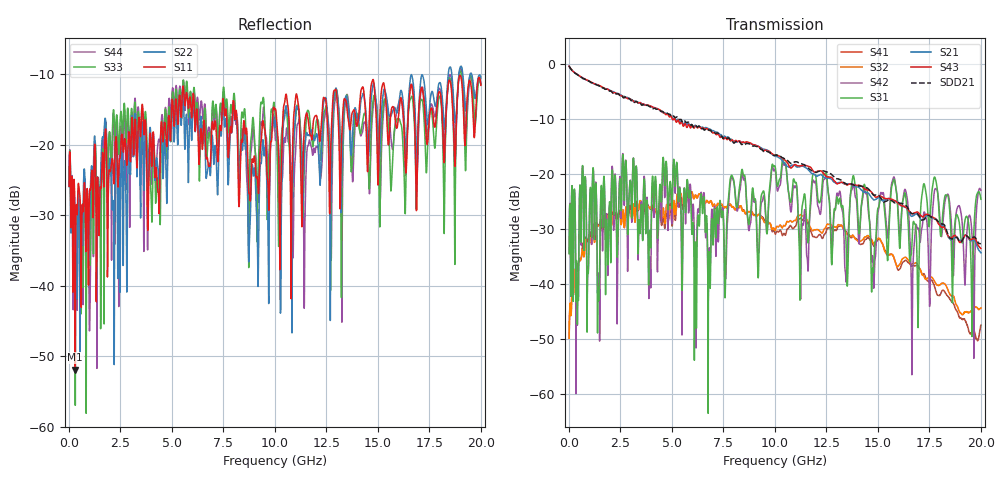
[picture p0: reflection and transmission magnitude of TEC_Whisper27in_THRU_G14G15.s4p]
! Tyco Electronics
! G14G15_THRU
!! PART DESCRIPTION: Whisper 27in Megtron 6 VLP-HVLP-VLP Channel Model, bulkhead 2.4mm test pts
!! MODEL DESCRIPTION: System 4-port S-parameter
!! MODEL STATUS: Measured
!! MODEL GEOMETRY: Channel Model
!! MODEL FREQUENCY RANGE: DC to 20.000 GHz in 10.000 MHz frequency steps
!! MODEL EDGE RATE LIMITATION: 25.00 ps (Using conservative 0.5/Fmax rule of thumb)
!! TIME-DOMAIN TRANSFORM CAUTIONS:
!! 1.) Do not simulate transient edge rates faster than the number listed above.  Edge rates faster than this number
!!  contain significant spectral content at frequencies above the model's highest frequency.
!! 2.) Even when simulating edge rates that are slower than the number listed above, be aware that the best time
!!  resolution possible with a direct iFFT is (1 / 2Fmax).  As a result, time resolution is typically not adequate
!!  for most time-domain simulations unless tricks such as windowing are used to minimize leakage and aliasing.
!! 3.) Because the model has a uniform frequency step, a direct iFFT will result in an impulse that that has a time
!!  length given by either (1 / Fstep) or (1 / 2Fstep), depending on the transform being used.  Care has been taken
!!  in selecting the frequency step to ensure a settled impulse response for the model.  Therefore, convolution with
!!  the model's impulse response should present no issues.  However, if directly concatenating s-parameter models
!!  in the frequency domain a user must either interpolate necessary interim frequencies or complete impulse response
!!  zero-padding.  Impulse response zero-padding is more difficult, but more accurate.
!! PORT DEFINITIONS:
!! Port  1  ----->  Side A  G14  Side B  <-----  Port  2
!! Port  3  ----->  Side A  G15  Side B  <-----  Port  4
! Point-to-Point link (differential)  !
! Connectors:  !
!  1: STRADA Whisper  !
! Materials:  !
!  Backplane: Megtron-6 HVLP  !
!  Daughtercard: Megtron-6 VLP  !
! Stack-up:  !
!  Backplane: 20 layers, 200mil thick  !
!  Daughtercard: 14 layers, 110mil thick  !
! Trace Length:  !
!  Backplane: 17in  !
!  Daightercards: 5in  !
! Trace Width:  !
!  Backplane: 8-13-8 mils  !
!  Daughtercards: 6-9-6 mils  !
! Geometry:  !
!  Backplane: Stripline  !
!  Daughtercards: Stripline  !
! Layer Connections:  !
!  Backplane: Layer 16, counterbored(1-6mil stub)  !
!  Daughtercard: Layer 9, counterbored(1-6mil stub) !
! Freq. Range: 0 GHz - 20 GHz  !
! Note1: non-mixed-mode s-parameters  !
! Note2: channel includes 2.4mm test points  !
! Created Wed May 11 14:53:33 2011
! 4 Port Network Data from SP1.SP block
! freq  magS11  angS11  magS12  angS12  magS13  angS13  magS14  angS14
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# hz S ma R 50
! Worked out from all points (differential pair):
!   2000 points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, 10 MHz to 20 GHz, reference 50 ohm
!   strongest paths, dB at 10 MHz, 5.01 GHz, 10.01 GHz, 15.01 GHz, 20 GHz:
!     S43: -0.4, -9.9, -16.5, -24.0, -33.5
!     S21: -0.4, -9.7, -16.7, -24.3, -34.3
!     S31: -34.5, -25.3, -18.6, -26.1, -24.6
!     S42: -34.4, -27.8, -19.1, -26.8, -22.9
!     S32: -49.8, -28.5, -30.2, -31.7, -44.3
!     S41: -49.8, -29.4, -30.9, -31.9, -47.4
!   taken as a pair (ports 3,1 in; 4,2 out), SDD21 dB: -0.3, -9.6, -16.6, -23.8, -32.7
!   lowest |S11| = -51.9 dB at 310 MHz (marker M1), VSWR 1.01, Z = 50 + j0.252 ohm
!   |S11| at or under -10 dB: start of sweep to end of sweep
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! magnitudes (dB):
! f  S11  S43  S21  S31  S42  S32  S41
! 10 MHz  -25.8  -0.4  -0.4  -34.5  -34.4  -49.8  -49.8
! 310 MHz  -51.9  -1.6  -1.6  -28.5  -28.9  -37.6  -37.5
! 5.88 GHz  -13.2  -11.5  -11.1  -23.0  -21.8  -23.6  -23.6
! 10.25 GHz  -36.2  -16.8  -17.1  -20.8  -22.0  -29.2  -30.2
! 15.77 GHz  -14.8  -24.7  -24.9  -21.0  -20.5  -35.1  -35.0
! 16.67 GHz  -12.0  -27.2  -27.6  -31.3  -44.7  -36.3  -36.7
! 20 GHz  -11.5  -33.5  -34.3  -24.6  -22.9  -44.3  -47.4
